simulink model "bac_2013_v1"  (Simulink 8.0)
settings: Solver=ode23t  StartTime=0.0  StopTime=150  RelTol=1e-5
libraries: fl_lib x10, nesl_utility x5, sdl_lib x2, elec_lib x1

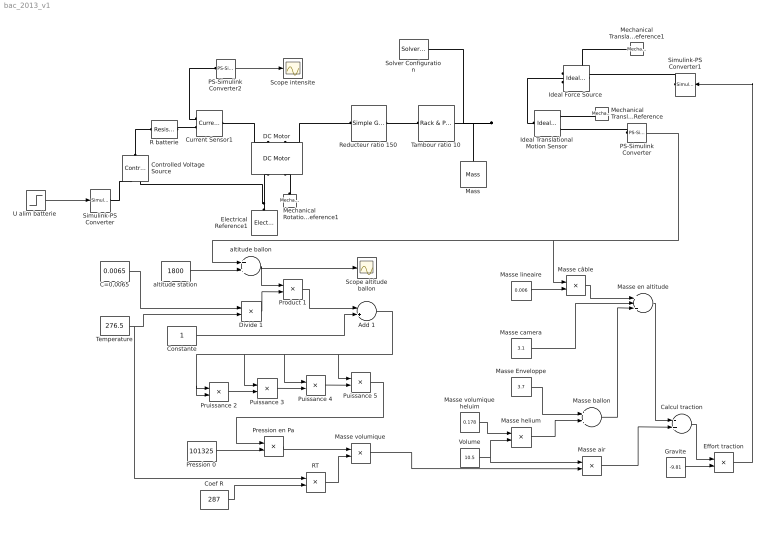
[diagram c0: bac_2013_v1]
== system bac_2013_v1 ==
  Add 1 : Sum  Inputs=-+
  C=0,0065 : Constant  Value=0.0065
  Calcul traction : Sum  Inputs=-+
  Coef R : Constant  Value=287
  Constante : Constant
  Controlled Voltage Source : fl_lib/Electrical/Electrical Sources/Controlled Voltage Source  i_Log=off  v_Log=off  LocalVarNames=|i|v  LocalVarDescs=|i|v  LocalVarLogging=[0 0]
  Current Sensor1 : fl_lib/Electrical/Electrical Sensors/Current Sensor  i1_Log=off  v1_Log=off  LocalVarNames=|i1|v1  LocalVarDescs=|i1|v1  LocalVarLogging=[0 0]
  DC Motor : elec_lib/Actuators & Drivers/Rotational Actuators/DC Motor  parameterization=1  Ra=.2 Ohm  La=1e-5 H  emf_or_torque=1  Kv=0.008 V/(rad/s)  Ki=6.876e-4 N*m/A  T_stall=2.4e-4 N*m  w_max=1.91e+4 rpm  w_rated=1.5e+4 rpm  P_rated=0.08 W  V_rated=1.5 V  J=4e-5 kg*m^2  lam_param=1  lam=0 N*m/(rad/s)  i_noload=0 A  V_i_noload=1.5 V  speed0=0 rpm  current_Log=off  voltage_Log=off  power_Log=off  i2r_Log=off  torque_Log=off  speed_Log=off  LocalVarNames=|current|voltage|power|i2r|torque|speed  LocalVarDescs=|Current (A)|Voltage (V)|Power (W)|Electrical losses (W)|Torque (Nm)|Angular speed (rad/s)  LocalVarLogging=[0 0 0 0 0 0]  alpha=0.00393 1/K  Tmeas=25 C  thermal_mass=100 J/K  initial_temperature=25 C
  Divide 1 : Product  Inputs=*/
  Effort traction : Product
  Electrical Reference1 : fl_lib/Electrical/Electrical Elements/Electrical Reference  i_Log=off  LocalVarNames=|i  LocalVarDescs=|i  LocalVarLogging=0
  Gravite : Constant  Value=-9.81
  Ideal Force Source : fl_lib/Mechanical/Mechanical Sources/Ideal Force Source  v_Log=off  f_Log=off  LocalVarNames=|v|f  LocalVarDescs=|v|f  LocalVarLogging=[0 0]
  Ideal Translational Motion Sensor : fl_lib/Mechanical/Mechanical Sensors/Ideal Translational Motion Sensor  offset=150 m  v_Log=off  f_Log=off  x_Log=off  LocalVarNames=|v|f|x  LocalVarDescs=|v|f|x  LocalVarLogging=[0 0 0]
  Mass : fl_lib/Mechanical/Translational Elements/Mass  mass=8.5 kg  initial_velocity=0 m/s  f_Log=off  LocalVarNames=|f  LocalVarDescs=|f  LocalVarLogging=0
  Masse Enveloppe : Constant  Value=3.7
  Masse air : Product
  Masse ballon : Sum
  Masse camera : Constant  Value=3.1
  Masse câble : Product
  Masse en altitude : Sum  Inputs=+++
  Masse helium : Product
  Masse lineaire : Constant  Value=0.006
  Masse volumique : Product  Inputs=*/
  Masse volumique heluim : Constant  Value=0.178
  Mechanical Rotational Reference1 : fl_lib/Mechanical/Rotational Elements/Mechanical Rotational Reference  t_Log=off  LocalVarNames=|t  LocalVarDescs=|t  LocalVarLogging=0
  Mechanical Translational Reference : fl_lib/Mechanical/Translational Elements/Mechanical Translational Reference  f_Log=off  LocalVarNames=|f  LocalVarDescs=|f  LocalVarLogging=0
  Mechanical Translational Reference1 : fl_lib/Mechanical/Translational Elements/Mechanical Translational Reference  f_Log=off  LocalVarNames=|f  LocalVarDescs=|f  LocalVarLogging=0
  PS-Simulink Converter : nesl_utility/PS-Simulink Converter  PhysicalDomain=network_engine_domain  LeftPortType=input  RightPortType=output  SubClassName=ps_output  PseudoPeriodic=off  Frequencies=[]  Unit=m  AffineConversion=off
  PS-Simulink Converter2 : nesl_utility/PS-Simulink Converter  PhysicalDomain=network_engine_domain  LeftPortType=input  RightPortType=output  SubClassName=ps_output  PseudoPeriodic=off  Frequencies=[]  Unit=A  AffineConversion=off
  Pression 0 : Constant  Value=101325
  Pression en Pa : Product
  Product 1 : Product
  Pruissance 2 : Product
  Puissance 3 : Product
  Puissance 4 : Product
  Puissance 5 : Product
  R batterie : fl_lib/Electrical/Electrical Elements/Resistor  R=0.13 Ohm  i_Log=off  v_Log=off  LocalVarNames=|i|v  LocalVarDescs=|i|v  LocalVarLogging=[0 0]
  RT : Product
  Reducteur ratio 150 : sdl_lib/Gears/Simple Gear  ratio=150  rotation_direction=2  friction_model=2  T_noload=0.1 N*m  T_nom=5 N*m  efficiency_nom=0.8  efficiency=0.6  mu_visc=[ 0 0 ] N*m/(rad/s)  w_thr=0.01 rad/s  LocalVarLogging=[]
  Scope altitude ballon : Scope
  Scope intensite : Scope
  Simulink-PS Converter : nesl_utility/Simulink-PS Converter  PhysicalDomain=network_engine_domain  LeftPortType=input  RightPortType=output  SubClassName=ps_input  PseudoPeriodic=off  Frequencies=[]  NoiseDistribution=none  NoiseParameters=[]  Unit=V  AffineConversion=off  InputFilterTimeConstant=.001  UdotUserProvided=1  SimscapeFilterOrder=1  InputFiltering=off
  Simulink-PS Converter1 : nesl_utility/Simulink-PS Converter  PhysicalDomain=network_engine_domain  LeftPortType=input  RightPortType=output  SubClassName=ps_input  PseudoPeriodic=off  Frequencies=[]  NoiseDistribution=none  NoiseParameters=[]  Unit=N  AffineConversion=off  InputFilterTimeConstant=.001  UdotUserProvided=1  SimscapeFilterOrder=1  InputFiltering=off
  Solver Configuration : nesl_utility/Solver Configuration  PhysicalDomain=network_engine_domain  LeftPortType=input  RightPortType=generic  SubClassName=solver  Accelerate=off  Profile=off  UseLocalSampling=off  FrequencyDomain=off  Tones=[]  Harmonics=[]  UseCCode=off  SimulateNoise=off  EnableSwitchedLinearOptims=on  DoDC=off  ResidualTolerance=1e-9  UseLocalSolver=off  LocalSolverChoice=NE_BACKWARD_EULER_ADVANCER  LocalSolverSampleTime=.001  DoFixedCost=off  MaxNonlinIter=3  MaxModeIter=2  LinearAlgebra=Sparse  DelaysMemoryBudget=1024
  Tambour ratio 10 : sdl_lib/Gears/Rotational- Translational/Rack & Pinion  param=1  radius=100 mm  n_teeth=20  x_tooth=5 mm  rack_direction_sign=1  friction_model=1  efficiency=0.8  mu_visc_P=0 N*m/(rad/s)  mu_visc_R=0 N/(m/s)  v_thr=0.001 m/s  LocalVarLogging=[]
  Temperature : Constant  Value=276.5
  "U alim batterie " : Step  Time=0  After=12  SampleTime=0
  Volume : Constant  Value=10.5
  altitude ballon : Sum
  altitude station : Constant  Value=1800
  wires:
  Masse câble/1 -> Masse en altitude/1
  Masse camera/1 -> Masse en altitude/2
  Masse volumique heluim/1 -> Masse helium/1
  Volume/1 -> Masse helium/2, Masse air/1
  Masse helium/1 -> Masse ballon/2
  Masse Enveloppe/1 -> Masse ballon/1
  Masse ballon/1 -> Masse en altitude/3
  Masse en altitude/1 -> Calcul traction/1
  Masse air/1 -> Calcul traction/2
  Calcul traction/1 -> Effort traction/1
  Gravite/1 -> Effort traction/2
  Effort traction/1 -> Simulink-PS Converter1/1
  PS-Simulink Converter2/1 -> Scope intensite/1
  PS-Simulink Converter/1 -> altitude ballon/1, Masse câble/1
  Divide 1/1 -> Product 1/2
  Puissance 3/1 -> Puissance 4/2
  Product 1/1 -> Add 1/1
  C=0,0065/1 -> Divide 1/1
  Puissance 4/1 -> Puissance 5/2
  Pruissance 2/1 -> Puissance 3/2
  Puissance 5/1 -> Pression en Pa/1
  Temperature/1 -> Divide 1/2, RT/1
  Add 1/1 -> Pruissance 2/2, Pruissance 2/1, Puissance 3/1, Puissance 4/1, Puissance 5/1
  Pression 0/1 -> Pression en Pa/2
  Constante/1 -> Add 1/2
  Masse volumique/1 -> Masse air/2
  Coef R/1 -> RT/2
  altitude ballon/1 -> Product 1/1, Scope altitude ballon/1
  altitude station/1 -> altitude ballon/2
  "U alim batterie "/1 -> Simulink-PS Converter/1
  Masse lineaire/1 -> Masse câble/2
  Pression en Pa/1 -> Masse volumique/1
  RT/1 -> Masse volumique/2
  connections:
  Mechanical Translational Reference/LConn1 -- Ideal Translational Motion Sensor/RConn1
  PS-Simulink Converter/LConn1 -- Ideal Translational Motion Sensor/RConn3
  Simulink-PS Converter1/RConn1 -- Ideal Force Source/RConn1
  Electrical Reference1/LConn1 -- Controlled Voltage Source/RConn2 -- DC Motor/RConn1
  Reducteur ratio 150/LConn1 -- DC Motor/LConn2
  Mechanical Rotational Reference1/LConn1 -- DC Motor/RConn2
  Ideal Force Source/RConn2 -- Mechanical Translational Reference1/LConn1
  Ideal Force Source/LConn1 -- Ideal Translational Motion Sensor/LConn1 -- Mass/LConn1 -- Tambour ratio 10/RConn1 -- Solver Configuration/RConn1
  Tambour ratio 10/LConn1 -- Reducteur ratio 150/RConn1
  Controlled Voltage Source/LConn1 -- R batterie/LConn1
  Simulink-PS Converter/RConn1 -- Controlled Voltage Source/RConn1
  R batterie/RConn1 -- Current Sensor1/RConn2
  Current Sensor1/LConn1 -- DC Motor/LConn1
  Current Sensor1/RConn1 -- PS-Simulink Converter2/LConn1
